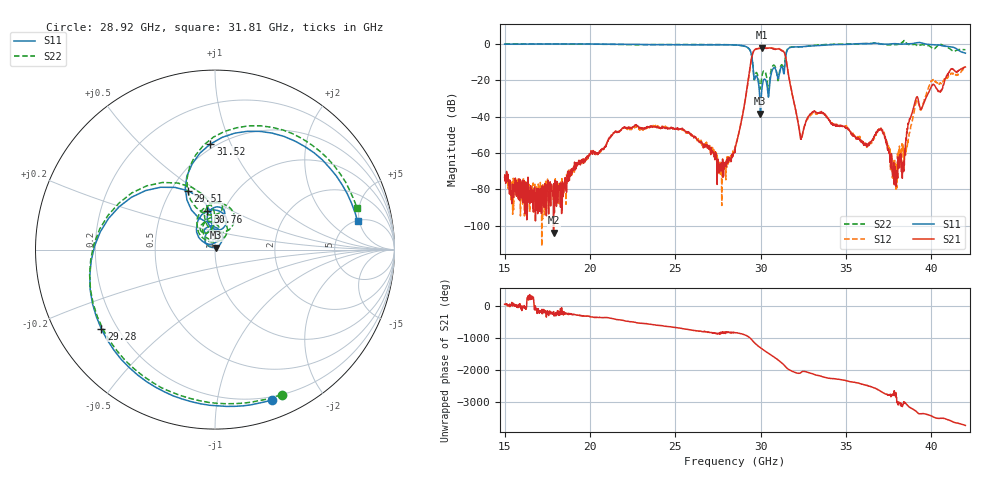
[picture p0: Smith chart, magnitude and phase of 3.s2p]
!The following data was pulled from an Agilent PNA
!This sNp file was generated from the data in the RF Test software
!NOTE:  Smoothing/Math/Corrections applied on any given trace ARE included in the data saved here
# MHz S dB R 50
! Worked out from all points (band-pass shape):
!   1601 points, 15 GHz to 42 GHz, reference 50 ohm
!   highest |S21| = -2.14 dB at 30.1 GHz (marker M1); lowest = -103.8 dB at 17.87 GHz (marker M2)
!   |S21| within 3 dB of the highest: 29.54 GHz to 31.4 GHz (1.864 GHz wide, 6.12 % of centre)
!   lowest |S11| = -38.3 dB at 29.98 GHz (marker M3), VSWR 1.02, Z = 50.4 + j1.15 ohm
!   |S11| at or under -10 dB: 29.53 GHz to 31.44 GHz (1.909 GHz wide, 6.26 % of centre)
!   |S22| runs from -27.3 to 1.9 dB; largest |S21 - S12| = 0.072
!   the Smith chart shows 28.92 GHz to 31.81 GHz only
!   S11 on the Smith chart (normalised r, x): 28.92 GHz: 0.17, -1.44; 29.28 GHz: 0.14, -0.31; 29.51 GHz: 0.61, +0.46; 30.76 GHz: 0.84, +0.38; 31.52 GHz: 0.47, +0.84; 31.81 GHz: 5.15, +4.70
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15000  -0.16 17.9  -73.37 56.6  -72.96 75.9  -0.13 18.6
17868.75  -0.07 -37.2  -103.75 -170.4  -86.41 147.1  -0.10 -36.6
19505.62  -0.08 -74.3  -65.29 57.9  -65.85 53.4  -0.14 -74.9
24011.25  -0.43 155.6  -46.09 117.5  -45.79 118.8  -0.39 152.3
26593.12  -0.54 73.0  -55.05 -78.4  -54.30 -75.6  -0.40 72.8
28500  -0.60 -21.3  -59.62 -106.1  -56.84 -109.0  -0.60 -17.3
28921.88  -0.96 -69.1  -40.31 -153.1  -39.86 -154.9  -1.03 -65.3
29276.25  -2.25 -145.2  -19.47 123.6  -20.19 121.9  -2.32 -144.5
29512.5  -8.86 114.6  -5.91 8.4  -6.16 12.0  -8.58 110.7
29985  -38.33 70.1  -2.36 139.9  -2.43 140.3  -24.27 114.3
30103.12  -22.72 139.1  -2.14 93.6  -2.34 95.5  -16.63 117.1
30390  -23.90 71.1  -2.46 -10.3  -2.32 -9.8  -20.69 52.1
30761.25  -13.28 101.1  -2.85 -145.1  -2.48 -144.8  -11.65 87.6
31081.88  -17.52 102.0  -2.84 92.9  -2.60 93.1  -16.98 107.6
31520.62  -4.60 92.5  -10.42 -131.7  -10.02 -133.1  -4.07 90.9
31807.5  -1.83 11.2  -25.30 134.0  -25.91 133.4  -1.67 16.1
32313.75  -1.62 -94.9  -49.65 65.5  -49.40 62.3  -1.70 -91.1
33005.62  -1.16 170.4  -37.80 50.3  -38.68 48.7  -0.99 167.6
37511.25  -0.12 24.9  -59.40 114.5  -59.84 118.1  -0.48 24.5
37899.38  0.10 17.5  -76.99 70.7  -78.45 -72.6  -0.40 21.7
39097.5  0.52 -1.4  -30.29 -42.4  -32.44 -26.4  -0.41 -4.0
42000  -5.11 -74.5  -12.70 -132.4  -13.38 -124.8  -3.21 -47.6
